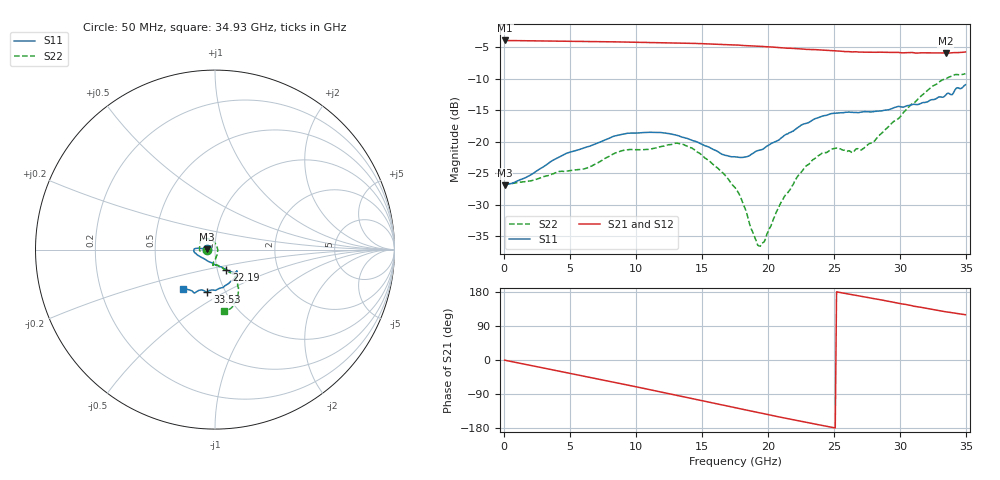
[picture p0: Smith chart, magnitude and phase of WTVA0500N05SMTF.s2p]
! 50 ohm 2-Port S-parameters measured by Modelithics Inc support@modelithics.com  Tampa, FL USA 813-866-6335 (February 2024)
! Smiths Interconnect,  5dB P/N: WTVA0500N05SMTF, Temperature: 75 C
! Board: 10 mil Rogers 4350B, Mounting Pad Dimensions: Length: 15 mils, Width: 25 mils, Gap: 40 mils.
# Hz S RI R 50
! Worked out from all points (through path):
!   352 points, 50 MHz to 34.93 GHz, reference 50 ohm
!   highest |S21| = -3.91 dB at 100 MHz (marker M1); lowest = -5.9 dB at 33.43 GHz (marker M2)
!   group delay of S21, straight-line fit = 19.5 ps
!   lowest |S11| = -26.9 dB at 50 MHz (marker M3), VSWR 1.09, Z = 45.7 + j0.0531 ohm
!   |S11| at or under -10 dB: start of sweep to end of sweep
!   |S22| runs from -36.6 to -9.2 dB; largest |S21 - S12| = 0.0065
!   S11 on the Smith chart (normalised r, x): 50 MHz: 0.91, +0.00; 22.19 GHz: 1.11, -0.25; 33.53 GHz: 0.82, -0.41; 34.93 GHz: 0.64, -0.31
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5e7  -0.045 0.00058  0.6374 -0.00362  0.6365 -0.00359  -0.0447 -0.00129
1e8  -0.0456 0.000144  0.6374 -0.00815  0.6366 -0.00823  -0.0458 -0.000832
2.986e9  -0.0627 0.00606  0.5905 -0.2275  0.5894 -0.2279  -0.0522 -0.00736
5.8715e9  -0.0874 0.00782  0.4703 -0.4157  0.4698 -0.4152  -0.0581 -0.0153
8.956e9  -0.1142 0.00444  0.2787 -0.5538  0.2777 -0.5531  -0.0846 -0.00637
1.1742e10  -0.1178 -0.0119  0.072 -0.6081  0.0707 -0.6074  -0.0846 0.0324
1.3135e10  -0.1103 -0.0188  -0.0359 -0.6075  -0.0373 -0.6065  -0.0801 0.055
1.42295e10  -0.0984 -0.0286  -0.1215 -0.5923  -0.1225 -0.5912  -0.0629 0.0627
1.7513e10  -0.0399 -0.0643  -0.3436 -0.4759  -0.3435 -0.475  -0.00509 0.0425
1.8309e10  -0.0192 -0.073  -0.3863 -0.4325  -0.3861 -0.4317  0.0053 0.0279
1.92045e10  0.00149 -0.0848  -0.4283 -0.3813  -0.4274 -0.3812  0.0134 0.00682
1.94035e10  0.00586 -0.0856  -0.4369 -0.3695  -0.4361 -0.3694  0.0147 0.00116
2.09955e10  0.0398 -0.0996  -0.4899 -0.2667  -0.4893 -0.2663  0.011 -0.0314
2.21895e10  0.0638 -0.1111  -0.5139 -0.1915  -0.5137 -0.1899  0.00313 -0.0522
2.33835e10  0.0858 -0.1218  -0.5276 -0.1147  -0.5268 -0.1148  -0.00838 -0.0713
2.49755e10  0.1078 -0.1286  -0.5283 -0.0125  -0.5276 -0.0115  -0.00962 -0.0876
2.7065e10  0.1238 -0.1195  -0.5046 0.1062  -0.5035 0.1077  0.0113 -0.0853
2.91545e10  0.1193 -0.1343  -0.4634 0.2201  -0.4605 0.2241  0.0658 -0.1156
3.1841e10  0.0714 -0.1916  -0.3732 0.3445  -0.3708 0.3456  0.1282 -0.2066
3.3433e10  -0.0377 -0.2313  -0.3061 0.402  -0.3029 0.4036  0.1085 -0.2954
3.35325e10  -0.0425 -0.2369  -0.3034 0.4045  -0.2999 0.4062  0.1083 -0.3006
3.49255e10  -0.1765 -0.2218  -0.255 0.4487  -0.2541 0.4481  0.0479 -0.3438
